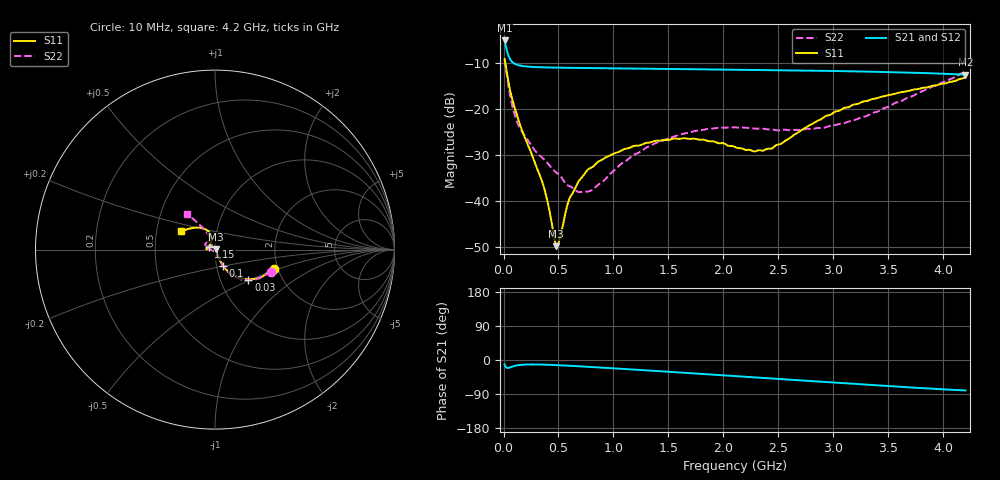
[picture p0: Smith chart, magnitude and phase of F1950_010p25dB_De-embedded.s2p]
! Integrated Device Technology
! Corporate Headquarters
! 6024 Silver Creek Valley Road
! San Jose, CA 95138  USA
! Phone:  1-408-284-8200
! Toll Free:  1-800-223-1366
! Webpage:  http://www.idt.com/
! Timing and RF Division
! 515 Groton Road, Suite 102
! Westford, MA 01886-6024
! Device:  F1950
! Description: 7-bit 0.25 dB Digital Step Attenuator
! Frequency:  150.0 -  4000.00 MHz
! Package:  4x4 mm Thin QFN Plastic Package: 24 pin
! Ports:  2 RF, 12 DC
!  Pin  1  = D0
!  Pin  2  = VDD
!  Pin  3  = Vmode
!  Pin  4  = GND
!  Pin  5  = RF1  =  Port 1
!  Pin  6  = GND
!  Pin  7  = GND
!  Pin  8  = GND
!  Pin  9  = GND
!  Pin 10  = GND
!  Pin 11  = GND
!  Pin 12  = GND
!  Pin 13  = GND
!  Pin 14  = RF2  =  Port 2
!  Pin 15  = GND
!  Pin 16  = LE
!  Pin 17  = CLK
!  Pin 18  = DATE
!  Pin 19  = D6
!  Pin 20  = D5
!  Pin 21  = D4
!  Pin 22  = D3
!  Pin 23  = D2
!  Pin 24  = D1
! State:  41
! Atten State:  10.25 dB
! Voltage:  +5.00 Volts
! Current:  Not Measured mA
! Data:  The device was measured on a the F195X evaluation board which has
!  individual transmission lines to the RF pins.  Data was collected
!  using a calibrated network analyzer.  The evaluation board was
!  de-embedded using a TRL calibration technique.
!  The reference plane is the edge of the package pin.
! Misc:  Board 2019
!  Action Tracker AT0250
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# GHz S dB R 50
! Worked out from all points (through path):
!   420 points, 10 MHz to 4.2 GHz, reference 50 ohm
!   highest |S21| = -5.20 dB at 10 MHz (marker M1); lowest = -12.6 dB at 4.2 GHz (marker M2)
!   group delay of S21, straight-line fit = 49.3 ps
!   lowest |S11| = -49.9 dB at 480 MHz (marker M3), VSWR 1.01, Z = 50.3 + j0.162 ohm
!   |S11| at or under -10 dB: 15.74 MHz to end of sweep
!   |S22| runs from -38.1 to -9.5 dB; largest |S21 - S12| = 0.00038
!   S11 on the Smith chart (normalised r, x): 10 MHz: 1.90, -0.46; 30 MHz: 1.36, -0.48; 100 MHz: 1.08, -0.20; 1.15 GHz: 0.93, +0.03; 4.2 GHz: 0.67, +0.15
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0.01  -9.25 -17.9  -5.20 -11.9  -5.20 -11.9  -9.47 -21.8
0.03  -12.05 -41.9  -7.34 -20.7  -7.34 -20.7  -12.88 -47.9
0.06  -16.01 -56.6  -9.27 -19.4  -9.27 -19.4  -17.19 -60.6
0.1  -19.68 -63.7  -10.23 -15.7  -10.23 -15.7  -21.21 -63.5
0.18  -25.47 -63.3  -10.77 -12.3  -10.77 -12.3  -25.44 -66.0
0.36  -36.49 -47.8  -11.04 -12.1  -11.04 -12.1  -30.80 -69.4
0.46  -47.84 -4.1  -11.09 -13.2  -11.09 -13.2  -33.47 -75.1
0.48  -49.85 30.0  -11.10 -13.4  -11.10 -13.4  -33.85 -77.6
0.51  -48.29 78.4  -11.11 -13.8  -11.11 -13.8  -34.41 -79.4
0.6  -39.50 117.1  -11.14 -15.2  -11.14 -15.2  -36.85 -93.9
0.71  -35.00 128.8  -11.18 -16.9  -11.18 -17.0  -38.07 -117.7
0.87  -31.41 140.1  -11.22 -19.7  -11.22 -19.7  -36.39 -155.6
1.15  -28.46 155.7  -11.30 -24.6  -11.30 -24.6  -30.62 175.2
1.41  -26.96 168.2  -11.36 -29.4  -11.36 -29.4  -27.22 166.2
1.73  -26.50 176.8  -11.44 -35.3  -11.44 -35.3  -24.90 158.0
2.11  -28.37 169.3  -11.55 -42.5  -11.54 -42.5  -24.11 147.9
2.28  -29.29 151.8  -11.59 -45.7  -11.59 -45.7  -24.33 142.3
2.43  -28.71 133.0  -11.64 -48.5  -11.64 -48.5  -24.51 136.9
2.81  -23.30 107.2  -11.76 -55.9  -11.76 -55.9  -24.42 120.4
3.1  -19.82 109.3  -11.87 -61.5  -11.87 -61.5  -23.12 114.7
3.51  -17.01 121.3  -12.07 -69.1  -12.07 -69.1  -19.50 115.9
4.2  -13.24 151.1  -12.64 -80.3  -12.64 -80.4  -11.94 127.9
